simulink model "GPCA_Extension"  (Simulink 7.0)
settings: Solver=ode45  StartTime=0.0  StopTime=inf  RelTol=1e-3
PreLoadFcn:
  | GPCA_Bus_Def
InitFcn:
  | script
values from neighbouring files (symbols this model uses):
  GOutputEvents = [0 0 0 0 0 0 0 0 0 0 0 0 0 0 0 0 0 0 0 0 0]    [script.m]
  GProgrammedDoseRate = 0    [script.m]
  GProgrammedVTBI = 0    [script.m]
undefined symbols (not defined in the file or in its folder): BarcodeReader, patientReader, y1, y2, y3, y4, y5, y6
libraries: simulink x3
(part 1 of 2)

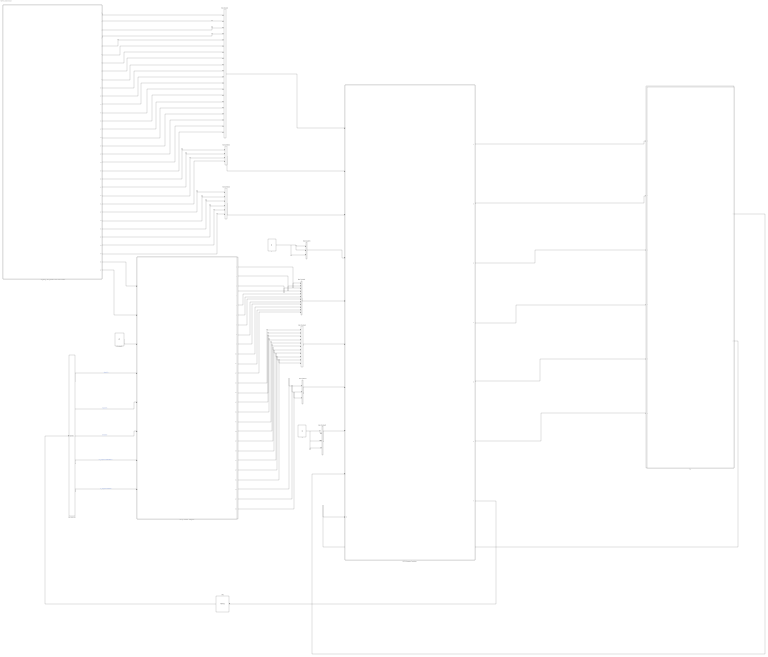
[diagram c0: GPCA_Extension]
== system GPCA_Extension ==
  1 : Constant  OutDataTypeMode=boolean  OutDataType=sfix(16)  OutScaling=2^0
  2 : Constant  Value=0  OutDataTypeMode=boolean  OutDataType=sfix(16)  OutScaling=2^0
  Bus Creator : BusCreator  Tag=DrugLIibraryInput  Description=Readings from the drug library  Inputs=20  UseBusObject=on
  Bus Creator1 : BusCreator  Description=Readings from the drug library  UseBusObject=on
  Bus Creator2 : BusCreator  Inputs=6  UseBusObject=on
  Bus Creator3 : BusCreator  Inputs=3  UseBusObject=on
  Bus Creator4 : BusCreator  Inputs=12  UseBusObject=on
  Bus Creator5 : BusCreator  Inputs=11  UseBusObject=on
  Bus Creator7 : BusCreator  Inputs=3  UseBusObject=on
  Bus Creator8 : BusCreator  Inputs=3  UseBusObject=on
  Bus Selector : BusSelector  OutputSignals=signal1,signal3,signal2,O_ProgrammedFlowRate,O_ProgrammedVTBI
  Constant5 : Constant  Value=0  OutDataType=sfix(16)  OutScaling=2^0
  Drug/Drug Library/Patient Information Reader : Subsystem
  GPCA Software Controller : Subsystem
  M2 : Memory  Orientation=left  InheritSampleTime=on
  Pump Controller Subsystem : Subsystem
  UI : Subsystem
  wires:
  Bus Creator/1 -> GPCA Software Controller/1(Drug Library Input)
  Bus Creator1/1 -> GPCA Software Controller/2(Patient Information Input)
  Bus Creator3/1 -> GPCA Software Controller/4(Environment Sensor Signals)
  Bus Creator4/1 -> GPCA Software Controller/5(Hardware Sensor Signals)
  Bus Creator7/1 -> GPCA Software Controller/7(Infusion Status Input)
  GPCA Software Controller/1(Drug Library Output) -> UI/1(Drug Lib)
  GPCA Software Controller/2(Patient Information Output) -> UI/2(Patient Info)
  GPCA Software Controller/4(Current State) -> UI/4(Current State)
  GPCA Software Controller/6(Alarming Condition) -> UI/6(Alarming Cond)
  GPCA Software Controller/3(Infusion Status Output) -> UI/3(Infusion Status)
  GPCA Software Controller/5(Drug Information Output) -> UI/5(Drug Info)
  1/1 -> Bus Creator8/1, Bus Creator8/2, Bus Creator8/3
  Bus Creator8/1 -> GPCA Software Controller/8(Pump Configuration Status Input)
  Bus Creator5/1 -> GPCA Software Controller/6(Infusion Sensor Signals)
  UI/2(Infusion Parameters) -> GPCA Software Controller/10(Infusion Parameters Input)
  UI/1(User Actions) -> GPCA Software Controller/9(User Actions)
  GPCA Software Controller/7(Infusion Instructions Output) -> M2/1
  Bus Selector/3 -> Pump Controller Subsystem/6(Infusion Paused)  "<signal2>"
  Bus Selector/2 -> Pump Controller Subsystem/5(Bolus Requested)  "<signal3>"
  Bus Selector/5 -> Pump Controller Subsystem/8(Programmed VTBI)  "<O_ProgrammedVTBI>"
  Bus Selector/1 -> Pump Controller Subsystem/4(Infusion In Progress)  "<signal1>"
  Bus Selector/4 -> Pump Controller Subsystem/7(Programmed Flow Rate)  "<O_ProgrammedFlowRate>"
  Constant5/1 -> Pump Controller Subsystem/3(New Bag Inserted)
  Drug/Drug Library/Patient Information Reader/32(Bolus Time) -> Pump Controller Subsystem/2(Bolus Time)
  Drug/Drug Library/Patient Information Reader/31(Bolus Volume) -> Pump Controller Subsystem/1(Bolus Volume)
  Bus Creator2/1 -> GPCA Software Controller/3(Drug Information Input)
  Drug/Drug Library/Patient Information Reader/30(drugVolumeUnit) -> Bus Creator2/6
  Drug/Drug Library/Patient Information Reader/29(drugDoseUnit) -> Bus Creator2/5
  Drug/Drug Library/Patient Information Reader/28(drugConcentration) -> Bus Creator2/4
  Drug/Drug Library/Patient Information Reader/27(drugDiluentVolume) -> Bus Creator2/3
  Drug/Drug Library/Patient Information Reader/26(drugDoseAmount) -> Bus Creator2/2
  Drug/Drug Library/Patient Information Reader/25(drugName) -> Bus Creator2/1
  Drug/Drug Library/Patient Information Reader/24(patientWeight) -> Bus Creator1/4
  Drug/Drug Library/Patient Information Reader/23(patientGender) -> Bus Creator1/3
  Drug/Drug Library/Patient Information Reader/22(patientAge) -> Bus Creator1/2
  Drug/Drug Library/Patient Information Reader/21(patientName) -> Bus Creator1/1
  Drug/Drug Library/Patient Information Reader/20(drugConcentrationLowerSoftLimit) -> Bus Creator/20
  Drug/Drug Library/Patient Information Reader/19(drugConcentrationLowerHardLimit) -> Bus Creator/19
  Drug/Drug Library/Patient Information Reader/18(drugConcentrationUpperSoftLimit) -> Bus Creator/18
  Drug/Drug Library/Patient Information Reader/17(drugConcentrationUpperHardLimit) -> Bus Creator/17
  Drug/Drug Library/Patient Information Reader/16(drugConcentrationTypical) -> Bus Creator/16
  Drug/Drug Library/Patient Information Reader/15(vtbiUnit) -> Bus Creator/15
  Drug/Drug Library/Patient Information Reader/14(vtbiLowerSoftLimit) -> Bus Creator/14
  Drug/Drug Library/Patient Information Reader/1(drugID) -> Bus Creator/1
  Drug/Drug Library/Patient Information Reader/2(amount) -> Bus Creator/2
  Drug/Drug Library/Patient Information Reader/3(diluentVolume) -> Bus Creator/3
  Drug/Drug Library/Patient Information Reader/4(doseRateTypical) -> Bus Creator/4
  Drug/Drug Library/Patient Information Reader/5(doseRateUpperHardLimit) -> Bus Creator/5
  Drug/Drug Library/Patient Information Reader/6(doseRateUpperSoftLimit) -> Bus Creator/6
  Drug/Drug Library/Patient Information Reader/7(doseRateLowerHardLimit) -> Bus Creator/7
  Drug/Drug Library/Patient Information Reader/8(doseRateLowerSoftLimit) -> Bus Creator/8
  Drug/Drug Library/Patient Information Reader/9(doseRateUnit) -> Bus Creator/9
  Drug/Drug Library/Patient Information Reader/10(vtbiTypical) -> Bus Creator/10
  Drug/Drug Library/Patient Information Reader/11(vtbiUpperHardLimit) -> Bus Creator/11
  Drug/Drug Library/Patient Information Reader/12(vtbiUpperSoftLimit) -> Bus Creator/12
  Drug/Drug Library/Patient Information Reader/13(vtbiLowerHardLimit) -> Bus Creator/13
  2/1 -> Bus Creator3/1, Bus Creator3/2, Bus Creator3/3
  Pump Controller Subsystem/1(Log Failure) -> Bus Creator4/1
  Pump Controller Subsystem/2(Watchdog Interrupt) -> Bus Creator4/2
  Pump Controller Subsystem/3(Door Open) -> Bus Creator4/3
  Pump Controller Subsystem/4(Battery Depleted) -> Bus Creator4/4
  Pump Controller Subsystem/5(Battery Low) -> Bus Creator4/5
  Pump Controller Subsystem/6(Battery Charge Error) -> Bus Creator4/6
  Pump Controller Subsystem/7(VoltOutRange) -> Bus Creator4/7
  Pump Controller Subsystem/8(CPU Error) -> Bus Creator4/8
  Pump Controller Subsystem/9(RTCError) -> Bus Creator4/9
  Pump Controller Subsystem/10(MemoryCorrupted) -> Bus Creator4/10
  Pump Controller Subsystem/11(PumpTooHot) -> Bus Creator4/11
  Pump Controller Subsystem/12(PumpOverheat) -> Bus Creator4/12
  Pump Controller Subsystem/13(EmptyReservoir) -> Bus Creator5/1
  Pump Controller Subsystem/14(LowReservoir) -> Bus Creator5/2
  Pump Controller Subsystem/15(Occlusion) -> Bus Creator5/3
  Pump Controller Subsystem/16(RateTooHigh) -> Bus Creator5/4
  Pump Controller Subsystem/17(RateTooLow) -> Bus Creator5/5
  Pump Controller Subsystem/18(LessThanKVO) -> Bus Creator5/6
  Pump Controller Subsystem/19(RateVary) -> Bus Creator5/7
  Pump Controller Subsystem/20(Flow Rate Above Pump Capacity Alarm) -> Bus Creator5/8
  Pump Controller Subsystem/21(PauseLong) -> Bus Creator5/9
  Pump Controller Subsystem/22(PauseTooLong) -> Bus Creator5/10
  Pump Controller Subsystem/23(Air In Line) -> Bus Creator5/11
  Pump Controller Subsystem/24(Bolus In Progress) -> Bus Creator7/1
  Pump Controller Subsystem/25(TotalVolumeInfused) -> Bus Creator7/2
  Pump Controller Subsystem/26(Current Volume) -> Bus Creator7/3
  M2/1 -> Bus Selector/1

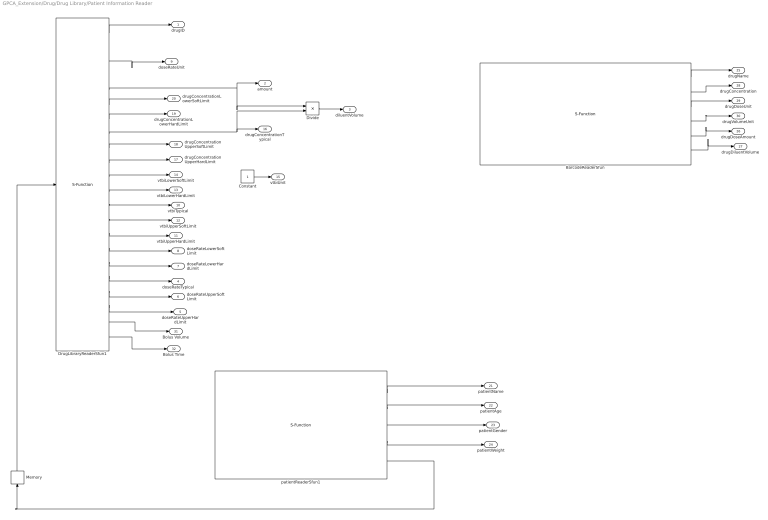
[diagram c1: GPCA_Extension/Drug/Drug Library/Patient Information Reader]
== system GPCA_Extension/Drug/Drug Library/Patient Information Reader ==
  BarcodeReaderSfun : S-Function  FunctionName=BarcodeReaderSfun  mask(Legacy Function){SFunctionSpec=BarcodeReader(uint32 y1[1], double y2[1], uint32 y3[1], uint32 y4[1], double y5[1], double y6[1]), ShowSpec=on}
      mask prompts: ShowSpec "Display function specification"
      mask help: This block allows the user to call the following C function(s) in Simulink: InitializeConditionsFcn: none StartFcn: openFile() OutputFcn: BarcodeReader(uint32 y1[1], double y2[1], uint32 y3[1], uint32 y4[1], double y5[1], double y6[1]) TerminateFcn: closeFile()
  Constant : Constant  OutDataTypeMode=uint32  OutDataType=sfix(16)  OutScaling=2^0
  Divide : Product  Inputs=*/  OutDataType=sfix(16)  OutScaling=2^-10
  DrugLibraryReaderSfun1 : S-Function  FunctionName=DrugLibraryReaderSfun  mask(Legacy Function){SFunctionSpec=DrugLibraryReader(uint32 u1[2], uint32 y1[1], uint32 y2[1], uint32 y3[1], uint32 y4[1], double  y5[1], double  y6[1], double  y7[1],double  y8[1],double  y9[1],double  y10[1],double  y11[1],double  y12[1], double  y13[1],double  y14[1],double  y15[1],double  y16[1],double  y17[1],double  y18[1],double  y19[1], double  y20[1],double  y21[1], uint32  y22[1]), ShowSpec=off}
      mask prompts: ShowSpec "Display function specification"
      mask help: This block allows the user to call the following C function(s) in Simulink: InitializeConditionsFcn: none StartFcn: openFile() OutputFcn: DrugLibraryReader(uint32 u1[2], uint32 y1[1], uint32 y2[1], uint32 y3[1], uint32 y4[1], double y5[1], double y6[1], double y7[1],double y8[1],double y9[1],double y10[1],double y11[1],double y12[1], double y13[1],double y14[1],double y15[1],double y16[1],double y17[1],double y18[1],double y19[1], double y20[1],double y21[1], uint32 y22[1]) TerminateFcn: closeFile()
  Memory : Memory  Orientation=up  InheritSampleTime=on
  patientReaderSfun1 : S-Function  FunctionName=patientReaderSfun  mask(Legacy Function){SFunctionSpec=patientReader(uint32 y1[1], uint32 y2[1], uint32 y3[1], uint32 y4[1], uint32 y5[2]), ShowSpec=on}
      mask prompts: ShowSpec "Display function specification"
      mask help: This block allows the user to call the following C function(s) in Simulink: InitializeConditionsFcn: randomizeSeed() StartFcn: openFile() OutputFcn: patientReader(uint32 y1[1], uint32 y2[1], uint32 y3[1], uint32 y4[1], uint32 y5[2]) TerminateFcn: closeFile()
  drugID : Outport  OutDataType=sfix(16)  OutScaling=2^0
  amount : Outport  Port=2  OutDataType=sfix(16)  OutScaling=2^0
  diluentVolume : Outport  Port=3  OutDataType=sfix(16)  OutScaling=2^0
  doseRateTypical : Outport  Port=4  OutDataType=sfix(16)  OutScaling=2^0
  doseRateUpperHardLimit : Outport  Port=5  OutDataType=sfix(16)  OutScaling=2^0
  doseRateUpperSoftLimit : Outport  Port=6  OutDataType=sfix(16)  OutScaling=2^0
  doseRateLowerHardLimit : Outport  Port=7  OutDataType=sfix(16)  OutScaling=2^0
  doseRateLowerSoftLimit : Outport  Port=8  OutDataType=sfix(16)  OutScaling=2^0
  doseRateUnit : Outport  Port=9  OutDataType=sfix(16)  OutScaling=2^0
  vtbiTypical : Outport  Port=10  OutDataType=sfix(16)  OutScaling=2^0
  vtbiUpperHardLimit : Outport  Port=11  OutDataType=sfix(16)  OutScaling=2^0
  vtbiUpperSoftLimit : Outport  Port=12  OutDataType=sfix(16)  OutScaling=2^0
  vtbiLowerHardLimit : Outport  Port=13  OutDataType=sfix(16)  OutScaling=2^0
  vtbiLowerSoftLimit : Outport  Port=14  OutDataType=sfix(16)  OutScaling=2^0
  vtbiUnit : Outport  Port=15  OutDataType=sfix(16)  OutScaling=2^0
  drugConcentrationTypical : Outport  Port=16  OutDataType=sfix(16)  OutScaling=2^0
  drugConcentrationUpperHardLimit : Outport  Port=17  OutDataType=sfix(16)  OutScaling=2^0
  drugConcentrationUpperSoftLimit : Outport  Port=18  OutDataType=sfix(16)  OutScaling=2^0
  drugConcentrationLowerHardLimit : Outport  Port=19  OutDataType=sfix(16)  OutScaling=2^0
  drugConcentrationLowerSoftLimit : Outport  Port=20  OutDataType=sfix(16)  OutScaling=2^0
  patientName : Outport  Port=21  OutDataType=sfix(16)  OutScaling=2^0
  patientAge : Outport  Port=22  OutDataType=sfix(16)  OutScaling=2^0
  patientGender : Outport  Port=23  OutDataType=sfix(16)  OutScaling=2^0
  patientWeight : Outport  Port=24  OutDataType=sfix(16)  OutScaling=2^0
  drugName : Outport  Port=25  OutDataType=sfix(16)  OutScaling=2^0
  drugDoseAmount : Outport  Port=26  OutDataType=sfix(16)  OutScaling=2^0
  drugDiluentVolume : Outport  Port=27  OutDataType=sfix(16)  OutScaling=2^0
  drugConcentration : Outport  Port=28  OutDataType=sfix(16)  OutScaling=2^0
  drugDoseUnit : Outport  Port=29  OutDataType=sfix(16)  OutScaling=2^0
  drugVolumeUnit : Outport  Port=30  OutDataType=sfix(16)  OutScaling=2^0
  Bolus Volume : Outport  Port=31  OutDataType=sfix(16)  OutScaling=2^0
  Bolus Time : Outport  Port=32  OutDataType=sfix(16)  OutScaling=2^0
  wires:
  patientReaderSfun1/5 -> Memory/1
  Memory/1 -> DrugLibraryReaderSfun1/1
  Divide/1 -> diluentVolume/1
  Constant/1 -> vtbiUnit/1
  patientReaderSfun1/1 -> patientName/1
  patientReaderSfun1/2 -> patientAge/1
  patientReaderSfun1/3 -> patientGender/1
  patientReaderSfun1/4 -> patientWeight/1
  BarcodeReaderSfun/1 -> drugName/1
  BarcodeReaderSfun/2 -> drugConcentration/1
  BarcodeReaderSfun/3 -> drugDoseUnit/1
  BarcodeReaderSfun/4 -> drugVolumeUnit/1
  BarcodeReaderSfun/5 -> drugDoseAmount/1
  BarcodeReaderSfun/6 -> drugDiluentVolume/1
  DrugLibraryReaderSfun1/1 -> drugID/1
  DrugLibraryReaderSfun1/5 -> amount/1, Divide/1
  DrugLibraryReaderSfun1/6 -> drugConcentrationLowerSoftLimit/1
  DrugLibraryReaderSfun1/7 -> drugConcentrationLowerHardLimit/1
  DrugLibraryReaderSfun1/8 -> drugConcentrationTypical/1, Divide/2
  DrugLibraryReaderSfun1/9 -> drugConcentrationUpperSoftLimit/1
  DrugLibraryReaderSfun1/10 -> drugConcentrationUpperHardLimit/1
  DrugLibraryReaderSfun1/11 -> vtbiLowerSoftLimit/1
  DrugLibraryReaderSfun1/12 -> vtbiLowerHardLimit/1
  DrugLibraryReaderSfun1/13 -> vtbiTypical/1
  DrugLibraryReaderSfun1/14 -> vtbiUpperSoftLimit/1
  DrugLibraryReaderSfun1/15 -> vtbiUpperHardLimit/1
  DrugLibraryReaderSfun1/16 -> doseRateLowerSoftLimit/1
  DrugLibraryReaderSfun1/17 -> doseRateLowerHardLimit/1
  DrugLibraryReaderSfun1/18 -> doseRateTypical/1
  DrugLibraryReaderSfun1/19 -> doseRateUpperSoftLimit/1
  DrugLibraryReaderSfun1/20 -> doseRateUpperHardLimit/1
  DrugLibraryReaderSfun1/3 -> doseRateUnit/1
  DrugLibraryReaderSfun1/21 -> Bolus Volume/1
  DrugLibraryReaderSfun1/22 -> Bolus Time/1

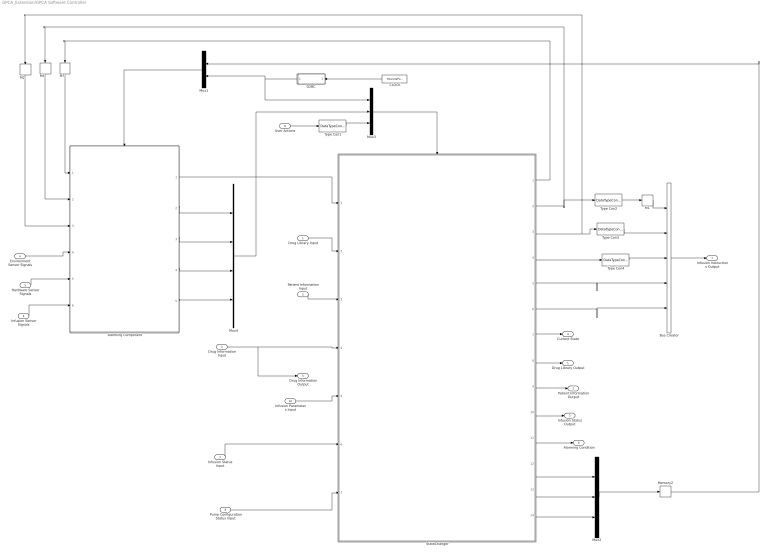
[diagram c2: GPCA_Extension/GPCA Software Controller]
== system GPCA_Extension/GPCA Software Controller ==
  Drug Library Input : Inport  OutDataType=sfix(16)  OutScaling=2^0
  Patient Information Input : Inport  Port=2  OutDataType=sfix(16)  OutScaling=2^0
  Drug Information Input : Inport  Port=3  OutDataType=sfix(16)  OutScaling=2^0
  Environment Sensor Signals : Inport  Port=4  OutDataType=sfix(16)  OutScaling=2^0
  Hardware Sensor Signals : Inport  Port=5  OutDataType=sfix(16)  OutScaling=2^0
  Infusion Sensor Signals : Inport  Port=6  OutDataType=sfix(16)  OutScaling=2^0
  Infusion Status Input : Inport  Port=7  OutDataType=sfix(16)  OutScaling=2^0
  Pump Configuration Status Input : Inport  Port=8  OutDataType=sfix(16)  OutScaling=2^0
  User Actions : Inport  Port=9  OutDataType=sfix(16)  OutScaling=2^0
  Infusion Parameters Input : Inport  Port=10  OutDataType=sfix(16)  OutScaling=2^0
  Alarming Component : Stateflow chart
  Bus Creator : BusCreator  Inputs=5  UseBusObject=on
  CLOCK : DiscretePulseGenerator  Orientation=left  PulseType=Time based  PulseWidth=50
  D2BC : Stateflow chart  Orientation=left
  M1 : Memory  InheritSampleTime=on
  M2 : Memory  Orientation=down  InheritSampleTime=on
  M4 : Memory  Orientation=down  InheritSampleTime=on
  M7 : Memory  Orientation=down  InheritSampleTime=on
  Memory2 : Memory  InheritSampleTime=on
  Mux1 : Mux  Orientation=left  Inputs=2
  Mux2 : Mux  Inputs=3
  Mux3 : Mux  Inputs=3
  Mux4 : Mux
  StateChanger : Stateflow chart
  Type Con1 : DataTypeConversion  OutDataTypeMode=boolean  OutDataType=sfix(16)  OutScaling=2^0
  Type Con2 : DataTypeConversion  OutDataType=sfix(16)  OutScaling=2^0
  Type Con3 : DataTypeConversion  OutDataType=sfix(16)  OutScaling=2^0
  Type Con4 : DataTypeConversion  OutDataType=sfix(16)  OutScaling=2^0
  Drug Library Output : Outport  OutDataType=sfix(16)  OutScaling=2^0
  Patient Information Output : Outport  Port=2  OutDataType=sfix(16)  OutScaling=2^0
  Infusion Status Output : Outport  Port=3  OutDataType=sfix(16)  OutScaling=2^0
  Current State : Outport  Port=4  OutDataType=sfix(16)  OutScaling=2^0
  Drug Information Output : Outport  Port=5  OutDataType=sfix(16)  OutScaling=2^0
  Alarming Condition : Outport  Port=6  OutDataType=sfix(16)  OutScaling=2^0
  Infusion Instructions Output : Outport  Port=7  OutDataType=sfix(16)  OutScaling=2^0
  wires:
  StateChanger/1(ClearCond) -> M7/1
  Mux3/1 -> StateChanger/Trigger
  Mux1/1 -> Alarming Component/Trigger
  StateChanger/2(O_InfusionInProgress) -> M4/1, Type Con2/1
  Alarming Component/1(ErrCond) -> StateChanger/1(ErrCond)
  User Actions/1 -> Type Con1/1
  StateChanger/12(E_Restart) -> Mux2/1
  StateChanger/13(E_AlarmClear) -> Mux2/2
  StateChanger/14(E_RequestToStart) -> Mux2/3
  Mux2/1 -> Memory2/1
  CLOCK/1 -> D2BC/1(u)
  D2BC/1(y) -> Mux1/2, Mux3/1
  Alarming Component/2(E_Alarm) -> Mux4/1
  Alarming Component/3(E_Warning) -> Mux4/2
  Alarming Component/4(E_Ready) -> Mux4/3
  Alarming Component/5(E_NotReady) -> Mux4/4
  Type Con1/1 -> Mux3/3
  Mux4/1 -> Mux3/2
  Type Con2/1 -> M1/1
  Memory2/1 -> Mux1/1
  Environment Sensor Signals/1 -> Alarming Component/4(envSenData)
  Hardware Sensor Signals/1 -> Alarming Component/5(hardwareSenData)
  Infusion Sensor Signals/1 -> Alarming Component/6(infuSenData)
  Drug Library Input/1 -> StateChanger/2(drugLibInfo)
  Patient Information Input/1 -> StateChanger/3(patientInfo)
  Drug Information Input/1 -> StateChanger/4(drugInfo), Drug Information Output/1
  Infusion Parameters Input/1 -> StateChanger/5(infuParameters)
  Infusion Status Input/1 -> StateChanger/6(infuStatus)
  Pump Configuration Status Input/1 -> StateChanger/7(pumpConfigData)
  StateChanger/11(O_AlarmCond) -> Alarming Condition/1
  StateChanger/7(O_CurrentState) -> Current State/1
  StateChanger/9(O_PatientInfo) -> Patient Information Output/1
  StateChanger/8(O_DrugLibInfo) -> Drug Library Output/1
  M1/1 -> Bus Creator/1
  StateChanger/3(O_InfusionPaused) -> M2/1, Type Con3/1
  Bus Creator/1 -> Infusion Instructions Output/1
  M7/1 -> Alarming Component/1(ClearCond)
  M4/1 -> Alarming Component/2(infusionInProgress)
  M2/1 -> Alarming Component/3(infusionPaused)
  StateChanger/4(O_BolusRequested) -> Type Con4/1
  StateChanger/5(O_ProgrammedVTBI) -> Bus Creator/4
  StateChanger/6(O_ProgrammedFlowRate) -> Bus Creator/5
  Type Con3/1 -> Bus Creator/2
  Type Con4/1 -> Bus Creator/3
  StateChanger/10(O_InfuStatus) -> Infusion Status Output/1

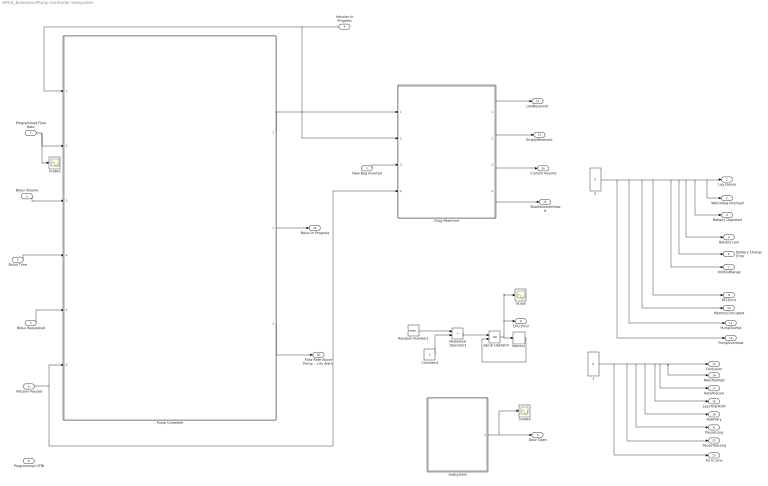
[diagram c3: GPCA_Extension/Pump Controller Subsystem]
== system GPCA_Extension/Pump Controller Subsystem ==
  Bolus Volume : Inport
  Bolus Time : Inport  Port=2
  New Bag Inserted : Inport  Port=3
  Infusion In Progress : Inport  Orientation=left  Port=4
  Bolus Requested : Inport  Port=5
  Infusion Paused : Inport  Port=6  OutDataType=sfix(16)  OutScaling=2^0
  Programmed Flow Rate : Inport  Port=7
  Programmed VTBI : Inport  Port=8
  1 : Constant  Value=0  OutDataTypeMode=boolean  OutDataType=sfix(16)  OutScaling=2^0
  2 : Constant  Value=0  OutDataTypeMode=boolean  OutDataType=sfix(16)  OutScaling=2^0
  Constant1 : Constant  Value=5  OutDataType=sfix(16)  OutScaling=2^0
  Drug Reservoir : Subsystem
  Logical Operator : Logic  Operator=OR  AllPortsSameDT=off  OutDataTypeMode=boolean
  Memory : Memory
  Pump Controller : Subsystem
  Random Number1 : RandomNumber  Mean=0.5
  Relational Operator1 : RelationalOperator  Operator=>  LogicOutDataTypeMode=boolean
  Scope : Scope
  Scope1 : Scope
  Scope2 : Scope
  Subsystem : Subsystem
  Log Failure : Outport  OutDataType=sfix(16)  OutScaling=2^0
  Watchdog Interrupt : Outport  Port=2  OutDataType=sfix(16)  OutScaling=2^0
  Door Open : Outport  Port=3  OutDataType=sfix(16)  OutScaling=2^0
  Battery Depleted : Outport  Port=4  OutDataType=sfix(16)  OutScaling=2^0
  Battery Low : Outport  Port=5  OutDataType=sfix(16)  OutScaling=2^0
  Battery Charge Error : Outport  Port=6  OutDataType=sfix(16)  OutScaling=2^0
  VoltOutRange : Outport  Port=7  OutDataType=sfix(16)  OutScaling=2^0
  CPU Error : Outport  Port=8  OutDataType=sfix(16)  OutScaling=2^0
  RTCError : Outport  Port=9  OutDataType=sfix(16)  OutScaling=2^0
  MemoryCorrupted : Outport  Port=10  OutDataType=sfix(16)  OutScaling=2^0
  PumpTooHot : Outport  Port=11  OutDataType=sfix(16)  OutScaling=2^0
  PumpOverheat : Outport  Port=12  OutDataType=sfix(16)  OutScaling=2^0
  EmptyReservoir : Outport  Port=13  OutDataType=sfix(16)  OutScaling=2^0
  LowReservoir : Outport  Port=14  OutDataType=sfix(16)  OutScaling=2^0
  Occlusion : Outport  Port=15  OutDataType=sfix(16)  OutScaling=2^0
  RateTooHigh : Outport  Port=16  OutDataType=sfix(16)  OutScaling=2^0
  RateTooLow : Outport  Port=17  OutDataType=sfix(16)  OutScaling=2^0
  LessThanKVO : Outport  Port=18  OutDataType=sfix(16)  OutScaling=2^0
  RateVary : Outport  Port=19  OutDataType=sfix(16)  OutScaling=2^0
  Flow Rate Above Pump Capacity Alarm : Outport  Port=20  OutDataType=sfix(16)  OutScaling=2^0
  PauseLong : Outport  Port=21  OutDataType=sfix(16)  OutScaling=2^0
  PauseTooLong : Outport  Port=22  OutDataType=sfix(16)  OutScaling=2^0
  Air In Line : Outport  Port=23  OutDataType=sfix(16)  OutScaling=2^0
  Bolus In Progress : Outport  Port=24  OutDataType=sfix(16)  OutScaling=2^0
  TotalVolumeInfused : Outport  Port=25  OutDataType=sfix(16)  OutScaling=2^0
  Current Volume : Outport  Port=26  OutDataType=sfix(16)  OutScaling=2^0
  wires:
  Bolus Requested/1 -> Pump Controller/5(Bolus Requested)
  Pump Controller/2(Bolus In Progress) -> Bolus In Progress/1
  Infusion Paused/1 -> Pump Controller/6(Infusion Paused), Drug Reservoir/4(Infusion Paused)
  New Bag Inserted/1 -> Drug Reservoir/3(New Bag Inserted)
  Drug Reservoir/3(Current Volume) -> Current Volume/1
  Drug Reservoir/2(DVA) -> EmptyReservoir/1
  Drug Reservoir/4(Total Volume Infused From Start) -> TotalVolumeInfused/1
  Infusion In Progress/1 -> Pump Controller/1(Infusion In Progress), Drug Reservoir/2(Infusion In Progress)
  Programmed Flow Rate/1 -> Pump Controller/2(Programmed Flow Rate), Scope1/1
  Drug Reservoir/1(LVW) -> LowReservoir/1
  Pump Controller/3(Flow Rate Above Pump Capacity Alarm) -> Flow Rate Above Pump Capacity Alarm/1
  Bolus Time/1 -> Pump Controller/4(Bolus Time)
  Bolus Volume/1 -> Pump Controller/3(Bolus Volume)
  2/1 -> RTCError/1, Battery Charge Error/1, Battery Low/1, Log Failure/1, Watchdog Interrupt/1, Battery Depleted/1, VoltOutRange/1, MemoryCorrupted/1, PumpTooHot/1, PumpOverheat/1
  1/1 -> RateTooLow/1, RateTooHigh/1, Occlusion/1, LessThanKVO/1, RateVary/1, PauseLong/1, PauseTooLong/1, Air In Line/1
  Pump Controller/1(Flow Rate) -> Drug Reservoir/1(Flow Rate)
  Random Number1/1 -> Relational Operator1/1
  Constant1/1 -> Relational Operator1/2
  Relational Operator1/1 -> Logical Operator/1
  Logical Operator/1 -> Memory/1, CPU Error/1, Scope/1
  Memory/1 -> Logical Operator/2
  Subsystem/1(Out1) -> Scope2/1, Door Open/1

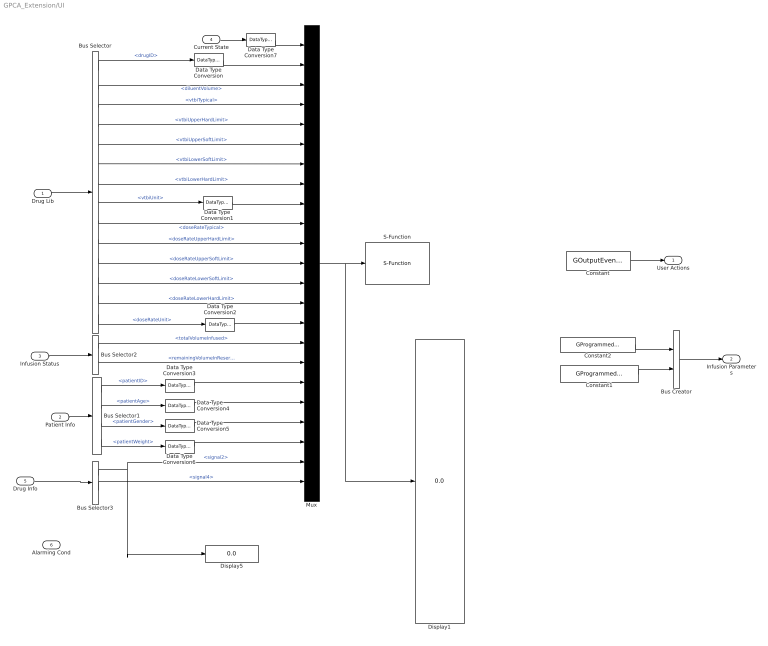
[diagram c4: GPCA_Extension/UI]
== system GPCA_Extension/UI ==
  Drug Lib : Inport  OutDataType=sfix(16)  OutScaling=2^0
  Patient Info : Inport  Port=2  OutDataType=sfix(16)  OutScaling=2^0
  Infusion Status : Inport  Port=3  OutDataType=sfix(16)  OutScaling=2^0
  Current State : Inport  Port=4  OutDataType=sfix(16)  OutScaling=2^0
  Drug Info : Inport  Port=5  OutDataType=sfix(16)  OutScaling=2^0
  Alarming Cond : Inport  Port=6  OutDataType=sfix(16)  OutScaling=2^0
  Bus Creator : BusCreator  Inputs=2  UseBusObject=on
  Bus Selector : BusSelector  OutputSignals=drugID,diluentVolume,vtbiTypical,vtbiUpperHardLimit,vtbiUpperSoftLimit,vtbiLowerSoftLimit,vtbiLowerHardLimit,vtbiUnit,doseRateTypical,doseRateUpperHardLimit,doseRateUpperSoftLimit,doseRateLowerSoftLimit,doseRateLowerHardLimit,doseRateUnit
  Bus Selector1 : BusSelector  OutputSignals=patientID,patientAge,patientGender,patientWeight
  Bus Selector2 : BusSelector  OutputSignals=totalVolumeInfused,remainingVolumeInReservoir
  Bus Selector3 : BusSelector  OutputSignals=signal2,signal4
  Constant : Constant  Value=GOutputEvents  OutDataType=sfix(16)  OutScaling=2^0
  Constant1 : Constant  Value=GProgrammedDoseRate  OutDataType=sfix(16)  OutScaling=2^0
  Constant2 : Constant  Value=GProgrammedVTBI  OutDataType=sfix(16)  OutScaling=2^0
  Data Type Conversion{,1..7} (8 alike) : DataTypeConversion  OutDataType=sfix(16)  OutScaling=2^0
  Display1 : Display
  Display5 : Display
  Mux : Mux  Inputs=23
  S-Function : S-Function  FunctionName=GPCA_UI_SFUN
  User Actions : Outport  OutDataType=sfix(16)  OutScaling=2^0
  Infusion Parameters : Outport  Port=2  OutDataType=sfix(16)  OutScaling=2^0
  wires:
  Current State/1 -> Data Type Conversion7/1
  Drug Lib/1 -> Bus Selector/1
  Bus Selector/1 -> Data Type Conversion/1  "<drugID>"
  Bus Selector/2 -> Mux/3  "<diluentVolume>"
  Bus Selector/3 -> Mux/4  "<vtbiTypical>"
  Bus Selector/4 -> Mux/5  "<vtbiUpperHardLimit>"
  Bus Selector/5 -> Mux/6  "<vtbiUpperSoftLimit>"
  Bus Selector/6 -> Mux/7  "<vtbiLowerSoftLimit>"
  Bus Selector/7 -> Mux/8  "<vtbiLowerHardLimit>"
  Bus Selector/8 -> Data Type Conversion1/1  "<vtbiUnit>"
  Bus Selector/9 -> Mux/10  "<doseRateTypical>"
  Bus Selector/10 -> Mux/11  "<doseRateUpperHardLimit>"
  Bus Selector/11 -> Mux/12  "<doseRateUpperSoftLimit>"
  Bus Selector/12 -> Mux/13  "<doseRateLowerSoftLimit>"
  Bus Selector/13 -> Mux/14  "<doseRateLowerHardLimit>"
  Bus Selector/14 -> Data Type Conversion2/1  "<doseRateUnit>"
  Patient Info/1 -> Bus Selector1/1
  Bus Selector1/1 -> Data Type Conversion3/1  "<patientID>"
  Bus Selector1/2 -> Data Type Conversion4/1  "<patientAge>"
  Bus Selector1/3 -> Data Type Conversion5/1  "<patientGender>"
  Bus Selector1/4 -> Data Type Conversion6/1  "<patientWeight>"
  Bus Selector3/1 -> Mux/22, Display5/1  "<signal2>"
  Bus Selector3/2 -> Mux/23  "<signal4>"
  Data Type Conversion/1 -> Mux/2
  Data Type Conversion1/1 -> Mux/9
  Data Type Conversion2/1 -> Mux/15
  Data Type Conversion3/1 -> Mux/18
  Data Type Conversion4/1 -> Mux/19
  Data Type Conversion5/1 -> Mux/20
  Data Type Conversion6/1 -> Mux/21
  Infusion Status/1 -> Bus Selector2/1
  Drug Info/1 -> Bus Selector3/1
  Constant/1 -> User Actions/1
  Constant2/1 -> Bus Creator/1
  Constant1/1 -> Bus Creator/2
  Bus Creator/1 -> Infusion Parameters/1
  Bus Selector2/1 -> Mux/16  "<totalVolumeInfused>"
  Bus Selector2/2 -> Mux/17  "<remainingVolumeInReservoir>"
  Data Type Conversion7/1 -> Mux/1
  Mux/1 -> S-Function/1, Display1/1

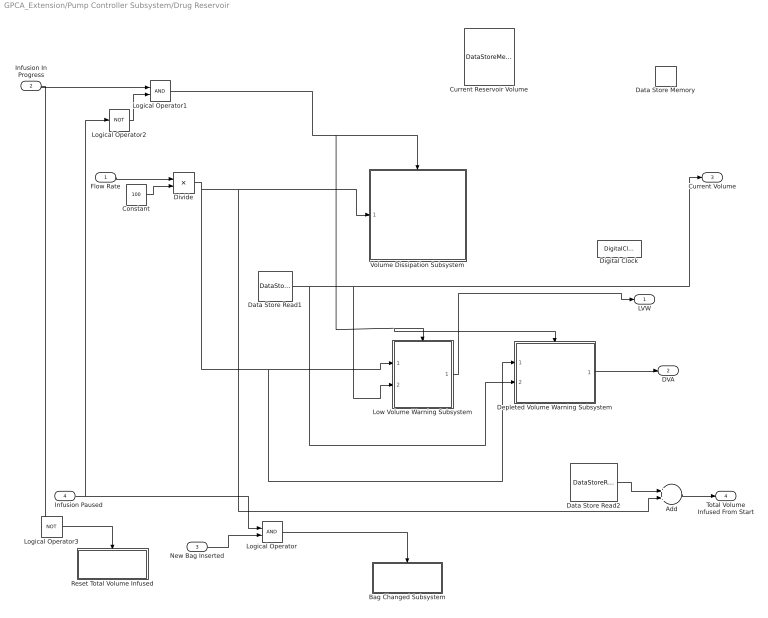
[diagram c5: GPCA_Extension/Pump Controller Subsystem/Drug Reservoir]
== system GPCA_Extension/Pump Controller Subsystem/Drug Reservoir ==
  Flow Rate : Inport
  Infusion In Progress : Inport  Port=2  OutDataType=sfix(16)  OutScaling=2^0
  New Bag Inserted : Inport  Port=3  OutDataType=sfix(16)  OutScaling=2^0
  Infusion Paused : Inport  Port=4  OutDataType=sfix(16)  OutScaling=2^0
  Add : Sum  OutDataType=sfix(16)  OutScaling=2^-10
  Bag Changed Subsystem : Subsystem  TreatAsAtomicUnit=on
  Constant : Constant  Value=100  OutDataType=sfix(16)  OutScaling=2^0
  Current Reservoir Volume : DataStoreMemory  DataStoreName=VolumeRes  InitialValue=2500  OutDataType=sfix(16)  OutScaling=2^0
  Data Store Memory : DataStoreMemory  DataStoreName=TVI  OutDataType=sfix(16)  OutScaling=2^0
  Data Store Read1 : DataStoreRead  DataStoreName=VolumeRes  SampleTime=-1
  Data Store Read2 : DataStoreRead  DataStoreName=TVI  SampleTime=-1
  Depleted Volume Warning Subsystem : Subsystem
  Digital Clock : DigitalClock
  Divide : Product  Inputs=*/  OutDataType=sfix(16)  OutScaling=2^-10
  Logical Operator : Logic  AllPortsSameDT=off  OutDataTypeMode=boolean
  Logical Operator1 : Logic  AllPortsSameDT=off  OutDataTypeMode=boolean
  Logical Operator2 : Logic  Operator=NOT  AllPortsSameDT=off  OutDataTypeMode=boolean
  Logical Operator3 : Logic  Operator=NOT  AllPortsSameDT=off  OutDataTypeMode=boolean
  Low Volume Warning Subsystem : Subsystem
  Reset Total Volume Infused : Subsystem  TreatAsAtomicUnit=on
  Volume Dissipation Subsystem : Subsystem
  LVW : Outport  OutDataType=sfix(16)  OutScaling=2^0
  DVA : Outport  Port=2  OutDataType=sfix(16)  OutScaling=2^0
  Current Volume : Outport  Port=3  OutDataType=sfix(16)  OutScaling=2^0
  Total Volume Infused From Start : Outport  Port=4  OutDataType=sfix(16)  OutScaling=2^0
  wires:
  Divide/1 -> Low Volume Warning Subsystem/1(Flow Rate), Depleted Volume Warning Subsystem/1(Flow Rate), Volume Dissipation Subsystem/1(Flow Rate), Add/2
  Logical Operator1/1 -> Volume Dissipation Subsystem/Enable, Low Volume Warning Subsystem/Enable, Depleted Volume Warning Subsystem/Enable
  Depleted Volume Warning Subsystem/1(DVA) -> DVA/1
  Low Volume Warning Subsystem/1(LVW) -> LVW/1
  Data Store Read1/1 -> Depleted Volume Warning Subsystem/2(Volume), Low Volume Warning Subsystem/2(Volume), Current Volume/1
  Infusion Paused/1 -> Logical Operator/1, Logical Operator2/1
  New Bag Inserted/1 -> Logical Operator/2
  Logical Operator/1 -> Bag Changed Subsystem/Enable
  Data Store Read2/1 -> Add/1
  Add/1 -> Total Volume Infused From Start/1
  Flow Rate/1 -> Divide/1
  Constant/1 -> Divide/2
  Infusion In Progress/1 -> Logical Operator1/1, Logical Operator3/1
  Logical Operator2/1 -> Logical Operator1/2
  Logical Operator3/1 -> Reset Total Volume Infused/Enable

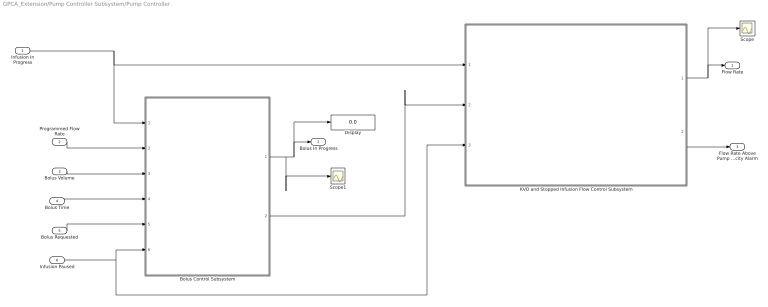
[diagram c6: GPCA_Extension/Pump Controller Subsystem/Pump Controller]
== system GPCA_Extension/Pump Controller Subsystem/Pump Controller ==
  Infusion In Progress : Inport  OutDataType=sfix(16)  OutScaling=2^0
  Programmed Flow Rate : Inport  Port=2  OutDataType=sfix(16)  OutScaling=2^0
  Bolus Volume : Inport  Port=3  OutDataType=sfix(16)  OutScaling=2^0
  Bolus Time : Inport  Port=4  OutDataType=sfix(16)  OutScaling=2^0
  Bolus Requested : Inport  Port=5  OutDataType=sfix(16)  OutScaling=2^0
  Infusion Paused : Inport  Port=6  OutDataType=sfix(16)  OutScaling=2^0
  Bolus Control Subsystem : Subsystem
  Display : Display
  KVO and Stopped Infusion Flow Control Subsystem : Subsystem
  Scope : Scope
  Scope1 : Scope
  Flow Rate : Outport
  Bolus In Progress : Outport  Port=2
  Flow Rate Above Pump Capacity Alarm : Outport  Port=3  OutDataType=sfix(16)  OutScaling=2^0
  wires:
  Infusion In Progress/1 -> KVO and Stopped Infusion Flow Control Subsystem/1(Infusion In Progress), Bolus Control Subsystem/1(Infusion In Progress)
  Programmed Flow Rate/1 -> Bolus Control Subsystem/2(Programmed Flow Rate)
  Bolus Requested/1 -> Bolus Control Subsystem/5(Bolus Requested)
  Bolus Volume/1 -> Bolus Control Subsystem/3(Bolus Volume)
  Bolus Time/1 -> Bolus Control Subsystem/4(Bolus Time)
  Bolus Control Subsystem/1(" Bolus In Progress") -> Scope1/1, Bolus In Progress/1, Display/1
  Infusion Paused/1 -> Bolus Control Subsystem/6(Infusion Paused), KVO and Stopped Infusion Flow Control Subsystem/3(Infusion Paused)
  Bolus Control Subsystem/2(Flow Rate) -> KVO and Stopped Infusion Flow Control Subsystem/2(Flow Rate from Bolus Subsystem)
  KVO and Stopped Infusion Flow Control Subsystem/1(Flow Rate) -> Flow Rate/1, Scope/1
  KVO and Stopped Infusion Flow Control Subsystem/2(" Flow Rate Above Pump Capacity Alarm") -> Flow Rate Above Pump Capacity Alarm/1

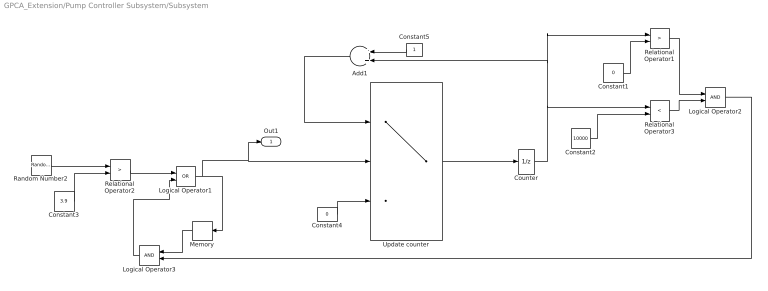
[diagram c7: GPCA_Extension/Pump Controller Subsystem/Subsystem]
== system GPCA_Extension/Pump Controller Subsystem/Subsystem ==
  Add1 : Sum  Orientation=left  OutDataType=sfix(16)  OutScaling=2^-10
  Constant1 : Constant  Value=0  OutDataType=sfix(16)  OutScaling=2^0
  Constant2 : Constant  Value=10000  OutDataType=sfix(16)  OutScaling=2^0
  Constant3 : Constant  Value=3.9  OutDataType=sfix(16)  OutScaling=2^0
  Constant4 : Constant  Value=0  OutDataType=sfix(16)  OutScaling=2^0
  Constant5 : Constant  Orientation=left  OutDataType=sfix(16)  OutScaling=2^0
  Counter : UnitDelay
  Logical Operator1 : Logic  Operator=OR  AllPortsSameDT=off  OutDataTypeMode=boolean
  Logical Operator2 : Logic  AllPortsSameDT=off  OutDataTypeMode=boolean
  Logical Operator3 : Logic  Orientation=left  AllPortsSameDT=off  OutDataTypeMode=boolean
  Memory : Memory  Orientation=left
  Random Number2 : RandomNumber  Mean=0.5
  Relational Operator1 : RelationalOperator  Operator=>  LogicOutDataTypeMode=boolean
  Relational Operator2 : RelationalOperator  Operator=>  LogicOutDataTypeMode=boolean
  Relational Operator3 : RelationalOperator  Operator=<  LogicOutDataTypeMode=boolean
  Update counter : Switch  Threshold=1  OutDataType=sfix(16)  OutScaling=2^0
  Out1 : Outport  OutDataType=sfix(16)  OutScaling=2^0
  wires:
  Random Number2/1 -> Relational Operator2/1
  Constant3/1 -> Relational Operator2/2
  Relational Operator2/1 -> Logical Operator1/1
  Logical Operator1/1 -> Memory/1, Update counter/2, Out1/1
  Add1/1 -> Update counter/1
  Constant5/1 -> Add1/1
  Counter/1 -> Relational Operator3/1, Add1/2, Relational Operator1/1
  Update counter/1 -> Counter/1
  Constant4/1 -> Update counter/3
  Constant2/1 -> Relational Operator3/2
  Relational Operator3/1 -> Logical Operator2/2
  Constant1/1 -> Relational Operator1/2
  Relational Operator1/1 -> Logical Operator2/1
  Memory/1 -> Logical Operator3/1
  Logical Operator2/1 -> Logical Operator3/2
  Logical Operator3/1 -> Logical Operator1/2

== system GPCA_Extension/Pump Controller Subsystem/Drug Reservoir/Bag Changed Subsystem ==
  Enable : EnablePort
  Constant : Constant  Value=10  OutDataType=sfix(16)  OutScaling=2^0
  Data Store Write : DataStoreWrite  DataStoreName=VolumeRes  SampleTime=-1
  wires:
  Constant/1 -> Data Store Write/1

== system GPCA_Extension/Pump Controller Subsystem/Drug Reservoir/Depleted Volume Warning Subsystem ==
  Flow Rate : Inport  OutDataType=sfix(16)  OutScaling=2^0
  Volume : Inport  Port=2  OutDataType=sfix(16)  OutScaling=2^0
  Enable : EnablePort
  Compare To Constant : simulink/Logic and Bit Operations/Compare To Constant  SystemSampleTime=-1  relop=<=  const=5  LogicOutDataTypeMode=boolean  ZeroCross=off
  Divide : Product  Inputs=*/  OutDataType=sfix(16)  OutScaling=2^-10
  DVA : Outport  OutDataType=sfix(16)  OutScaling=2^0
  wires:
  Volume/1 -> Divide/1
  Flow Rate/1 -> Divide/2
  Divide/1 -> Compare To Constant/1
  Compare To Constant/1 -> DVA/1

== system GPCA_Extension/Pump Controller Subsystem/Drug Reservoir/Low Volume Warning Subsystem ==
  Flow Rate : Inport  OutDataType=sfix(16)  OutScaling=2^0
  Volume : Inport  Port=2  OutDataType=sfix(16)  OutScaling=2^0
  Enable : EnablePort
  Compare To Constant : simulink/Logic and Bit Operations/Compare To Constant  SystemSampleTime=-1  relop=<=  const=15  LogicOutDataTypeMode=boolean  ZeroCross=off
  Compare To Constant1 : simulink/Logic and Bit Operations/Compare To Constant  SystemSampleTime=-1  relop=>  const=5  LogicOutDataTypeMode=boolean  ZeroCross=off
  Divide : Product  Inputs=*/  OutDataType=sfix(16)  OutScaling=2^-10
  Logical Operator : Logic  AllPortsSameDT=off  OutDataTypeMode=boolean
  LVW : Outport  OutDataType=sfix(16)  OutScaling=2^0
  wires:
  Volume/1 -> Divide/1
  Flow Rate/1 -> Divide/2
  Divide/1 -> Compare To Constant/1, Compare To Constant1/1
  Compare To Constant1/1 -> Logical Operator/2
  Compare To Constant/1 -> Logical Operator/1
  Logical Operator/1 -> LVW/1

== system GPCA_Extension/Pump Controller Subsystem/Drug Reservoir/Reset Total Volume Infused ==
  Enable : EnablePort
  Constant : Constant  Value=0  OutDataType=sfix(16)  OutScaling=2^0
  Data Store Write : DataStoreWrite  DataStoreName=TVI  SampleTime=-1
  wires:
  Constant/1 -> Data Store Write/1

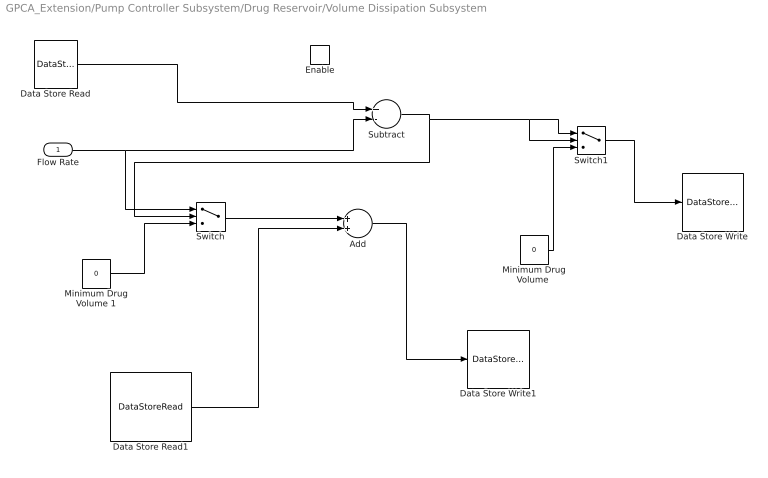
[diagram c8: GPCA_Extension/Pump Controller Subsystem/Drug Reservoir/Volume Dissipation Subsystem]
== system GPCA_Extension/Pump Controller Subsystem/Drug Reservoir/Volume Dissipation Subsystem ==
  Flow Rate : Inport  OutDataType=sfix(16)  OutScaling=2^0
  Enable : EnablePort
  Add : Sum  OutDataType=sfix(16)  OutScaling=2^-10
  Data Store Read : DataStoreRead  DataStoreName=VolumeRes  SampleTime=-1
  Data Store Read1 : DataStoreRead  DataStoreName=TVI  SampleTime=-1
  Data Store Write : DataStoreWrite  DataStoreName=VolumeRes  SampleTime=-1
  Data Store Write1 : DataStoreWrite  DataStoreName=TVI  SampleTime=-1
  "Minimum Drug Volume " : Constant  Value=0  OutDataTypeMode=double  OutDataType=sfix(16)  OutScaling=2^0
  Minimum Drug Volume 1 : Constant  Value=0  OutDataTypeMode=double  OutDataType=sfix(16)  OutScaling=2^0
  Subtract : Sum  Inputs=+-  OutDataType=sfix(16)  OutScaling=2^-10
  Switch : Switch  OutDataType=sfix(16)  OutScaling=2^0
  Switch1 : Switch  OutDataType=sfix(16)  OutScaling=2^0
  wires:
  Data Store Read/1 -> Subtract/1
  Flow Rate/1 -> Subtract/2, Switch/1
  Data Store Read1/1 -> Add/2
  Add/1 -> Data Store Write1/1
  Subtract/1 -> Switch/2, Switch1/1, Switch1/2
  Minimum Drug Volume 1/1 -> Switch/3
  Switch/1 -> Add/1
  "Minimum Drug Volume "/1 -> Switch1/3
  Switch1/1 -> Data Store Write/1

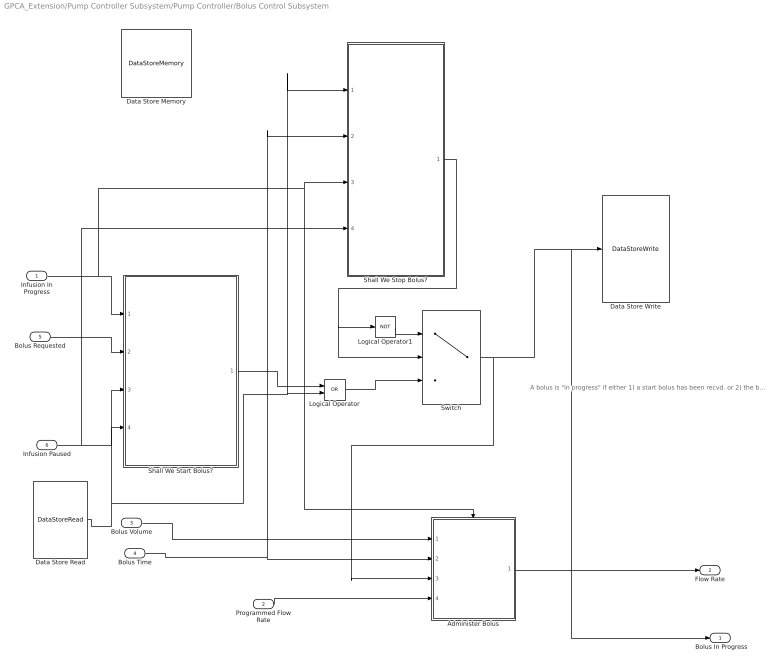
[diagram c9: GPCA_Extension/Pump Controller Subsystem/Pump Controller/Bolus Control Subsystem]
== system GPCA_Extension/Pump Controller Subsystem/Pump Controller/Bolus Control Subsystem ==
  note: A bolus is "in progress" if either 1) a start bolus has been recvd. or 2) the bolus was in progress in the preceeding simulation time. The only way a bolus that is in progress can become de-activated is if the bolus timer expires or if infusion is no longer in progress (can happen due to an alarm or user input). The switch block encodes this logic. As long as "Shall we Stop Bolus" outputs 0 (i.e. the bolus timer has not expired), the switch block outputs the value of "Start Bolus" OR "Bolus In Progress in Previous Step". As soon as "Shall We Stop Bolus" outputs 1, the switch outputs 0.
  Infusion In Progress : Inport  OutDataType=sfix(16)  OutScaling=2^0
  Programmed Flow Rate : Inport  Port=2  OutDataType=sfix(16)  OutScaling=2^0
  Bolus Volume : Inport  Port=3  OutDataType=sfix(16)  OutScaling=2^0
  Bolus Time : Inport  Port=4  OutDataType=sfix(16)  OutScaling=2^0
  Bolus Requested : Inport  Port=5  OutDataType=sfix(16)  OutScaling=2^0
  Infusion Paused : Inport  Port=6  OutDataType=sfix(16)  OutScaling=2^0
  Administer Bolus : Subsystem
  Data Store Memory : DataStoreMemory  DataStoreName=BolusInProgress  DataType=boolean  OutDataType=sfix(16)  OutScaling=2^0
  Data Store Read : DataStoreRead  DataStoreName=BolusInProgress  SampleTime=-1
  Data Store Write : DataStoreWrite  DataStoreName=BolusInProgress  SampleTime=-1
  Logical Operator : Logic  Operator=OR  AllPortsSameDT=off  OutDataTypeMode=boolean
  Logical Operator1 : Logic  Operator=NOT  AllPortsSameDT=off  OutDataTypeMode=boolean
  Shall We Start Bolus? : Subsystem
  Shall We Stop Bolus? : Subsystem
  Switch : Switch  Criteria=u2 ~= 0  OutDataType=sfix(16)  OutScaling=2^0
  " Bolus In Progress" : Outport  OutDataType=sfix(16)  OutScaling=2^0
  Flow Rate : Outport  Port=2  OutDataType=sfix(16)  OutScaling=2^0
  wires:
  Infusion In Progress/1 -> Shall We Start Bolus?/1(Infusion In Progress), Shall We Stop Bolus?/3(Infusion In Progress), Administer Bolus/Enable
  Bolus Requested/1 -> Shall We Start Bolus?/2(Bolus Requested)
  Data Store Read/1 -> Shall We Start Bolus?/3(Bolus In Progress), Logical Operator/2, Shall We Stop Bolus?/1(IsBolusInProgress)
  Bolus Volume/1 -> Administer Bolus/1(Bolus Volume)
  Bolus Time/1 -> Administer Bolus/2(Bolus Time), Shall We Stop Bolus?/2(Bolus Time)
  Programmed Flow Rate/1 -> Administer Bolus/4(Programmed Flow Rate)
  Administer Bolus/1(Out1) -> Flow Rate/1
  Switch/1 -> Administer Bolus/3(Bolus In Progress), Data Store Write/1, " Bolus In Progress"/1
  Shall We Start Bolus?/1(Start Bolus) -> Logical Operator/1
  Shall We Stop Bolus?/1(Stop Bolus) -> Switch/2, Logical Operator1/1
  Logical Operator1/1 -> Switch/1
  Infusion Paused/1 -> Shall We Start Bolus?/4(Infusion Paused), Shall We Stop Bolus?/4(Infusion Paused)
  Logical Operator/1 -> Switch/3

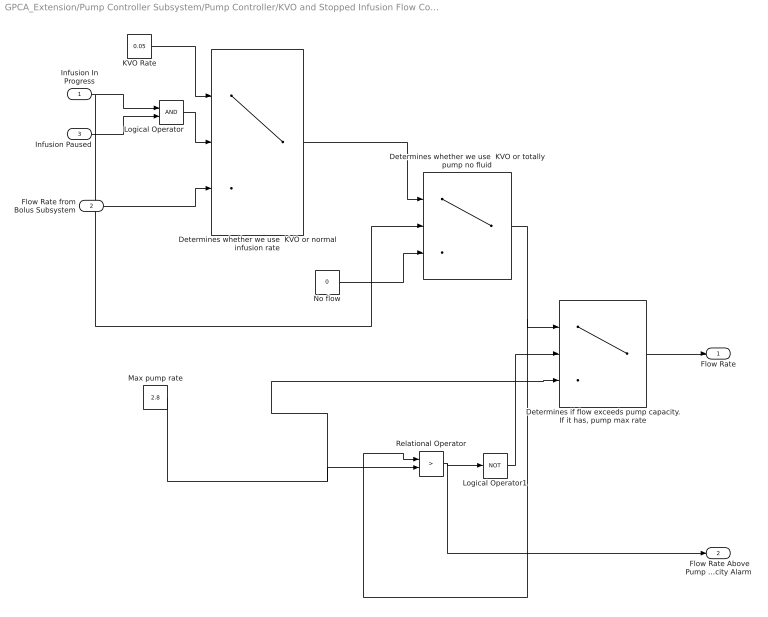
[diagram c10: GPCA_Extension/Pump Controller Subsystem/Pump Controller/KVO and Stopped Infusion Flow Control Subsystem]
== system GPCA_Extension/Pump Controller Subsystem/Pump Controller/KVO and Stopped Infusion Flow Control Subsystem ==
  Infusion In Progress : Inport
  Flow Rate from Bolus Subsystem : Inport  Port=2
  Infusion Paused : Inport  Port=3
  "Determines if flow exceeds pump capacity. If it has, pump max rate" : Switch  Criteria=u2 ~= 0  OutDataType=sfix(16)  OutScaling=2^0
  Determines whether we use  KVO or normal infusion rate : Switch  Criteria=u2 ~= 0  OutDataType=sfix(16)  OutScaling=2^0
  Determines whether we use  KVO or totally pump no fluid : Switch  Criteria=u2 ~= 0  OutDataType=sfix(16)  OutScaling=2^0
  KVO Rate : Constant  Value=0.05  OutDataType=sfix(16)  OutScaling=2^0
  Logical Operator : Logic  AllPortsSameDT=off  OutDataTypeMode=boolean
  Logical Operator1 : Logic  Operator=NOT  AllPortsSameDT=off  OutDataTypeMode=boolean
  Max pump rate : Constant  Value=2.8  OutDataType=sfix(16)  OutScaling=2^0
  No flow : Constant  Value=0  OutDataType=sfix(16)  OutScaling=2^0
  Relational Operator : RelationalOperator  Operator=>  LogicOutDataTypeMode=boolean
  Flow Rate : Outport
  " Flow Rate Above Pump Capacity Alarm" : Outport  Port=2  OutDataType=sfix(16)  OutScaling=2^0
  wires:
  KVO Rate/1 -> Determines whether we use  KVO or normal infusion rate/1
  Flow Rate from Bolus Subsystem/1 -> Determines whether we use  KVO or normal infusion rate/3
  Infusion In Progress/1 -> Logical Operator/1, Determines whether we use  KVO or totally pump no fluid/2
  Infusion Paused/1 -> Logical Operator/2
  Logical Operator/1 -> Determines whether we use  KVO or normal infusion rate/2
  Determines whether we use  KVO or normal infusion rate/1 -> Determines whether we use  KVO or totally pump no fluid/1
  No flow/1 -> Determines whether we use  KVO or totally pump no fluid/3
  "Determines if flow exceeds pump capacity. If it has, pump max rate"/1 -> Flow Rate/1
  Determines whether we use  KVO or totally pump no fluid/1 -> "Determines if flow exceeds pump capacity. If it has, pump max rate"/1, Relational Operator/1
  Max pump rate/1 -> "Determines if flow exceeds pump capacity. If it has, pump max rate"/3, Relational Operator/2
  Relational Operator/1 -> Logical Operator1/1, " Flow Rate Above Pump Capacity Alarm"/1
  Logical Operator1/1 -> "Determines if flow exceeds pump capacity. If it has, pump max rate"/2

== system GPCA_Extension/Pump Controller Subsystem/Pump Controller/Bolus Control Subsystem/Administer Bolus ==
  Bolus Volume : Inport  OutDataType=sfix(16)  OutScaling=2^0
  Bolus Time : Inport  Port=2  OutDataType=sfix(16)  OutScaling=2^0
  Bolus In Progress : Inport  Port=3
  Programmed Flow Rate : Inport  Port=4
  Enable : EnablePort
  Divide : Product  Inputs=*/  OutDataType=sfix(16)  OutScaling=2^-10
  Switch : Switch  Criteria=u2 ~= 0  OutDataType=sfix(16)  OutScaling=2^0
  Out1 : Outport
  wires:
  Bolus Volume/1 -> Divide/1
  Bolus Time/1 -> Divide/2
  Divide/1 -> Switch/1
  Bolus In Progress/1 -> Switch/2
  Switch/1 -> Out1/1
  Programmed Flow Rate/1 -> Switch/3

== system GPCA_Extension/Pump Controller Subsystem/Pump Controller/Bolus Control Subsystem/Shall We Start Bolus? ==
  Infusion In Progress : Inport  OutDataType=sfix(16)  OutScaling=2^0
  Bolus Requested : Inport  Port=2  OutDataType=sfix(16)  OutScaling=2^0
  Bolus In Progress : Inport  Port=3  OutDataType=sfix(16)  OutScaling=2^0
  Infusion Paused : Inport  Port=4  OutDataType=sfix(16)  OutScaling=2^0
  Logical Operator1 : Logic  Operator=NOT  AllPortsSameDT=off  OutDataTypeMode=boolean
  Logical Operator2 : Logic  Inputs=4  OutDataTypeMode=boolean
  Logical Operator3 : Logic  Operator=NOT  AllPortsSameDT=off  OutDataTypeMode=boolean
  Start Bolus : Outport  OutDataType=sfix(16)  OutScaling=2^0
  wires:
  Bolus Requested/1 -> Logical Operator2/2
  Bolus In Progress/1 -> Logical Operator1/1
  Infusion In Progress/1 -> Logical Operator2/1
  Logical Operator1/1 -> Logical Operator2/3
  Logical Operator2/1 -> Start Bolus/1
  Logical Operator3/1 -> Logical Operator2/4
  Infusion Paused/1 -> Logical Operator3/1

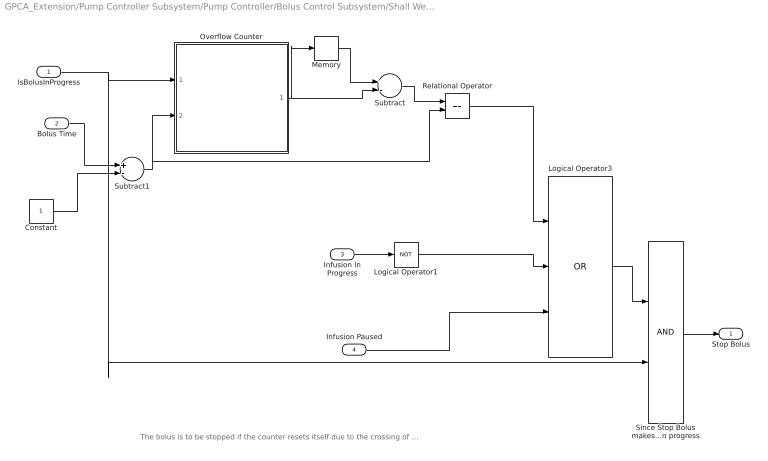
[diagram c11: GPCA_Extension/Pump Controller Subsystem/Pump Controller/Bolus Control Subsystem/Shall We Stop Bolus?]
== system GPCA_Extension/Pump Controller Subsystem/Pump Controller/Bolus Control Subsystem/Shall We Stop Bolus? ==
  note: The bolus is to be stopped if the counter resets itself due to the crossing of the upper limit. The memory block and the subtract block detects if the output of the counter fell from "Upper limit" to "zero"
  IsBolusInProgress : Inport
  Bolus Time : Inport  Port=2
  Infusion In Progress : Inport  Port=3  OutDataType=sfix(16)  OutScaling=2^0
  Infusion Paused : Inport  Port=4  OutDataType=sfix(16)  OutScaling=2^0
  Constant : Constant  OutDataType=sfix(16)  OutScaling=2^0
  Logical Operator1 : Logic  Operator=NOT  AllPortsSameDT=off  OutDataTypeMode=boolean
  Logical Operator3 : Logic  Operator=OR  Inputs=3  AllPortsSameDT=off  OutDataTypeMode=boolean
  Memory : Memory  InheritSampleTime=on
  Overflow Counter : Subsystem
  Relational Operator : RelationalOperator  Operator===  LogicOutDataTypeMode=boolean
  Since Stop Bolus makes sense only when there was bolus in progress : Logic  AllPortsSameDT=off  OutDataTypeMode=boolean
  Subtract : Sum  Inputs=+-  OutDataType=sfix(16)  OutScaling=2^-10
  Subtract1 : Sum  Inputs=+-  OutDataType=sfix(16)  OutScaling=2^-10
  Stop Bolus : Outport
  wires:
  Overflow Counter/1(Out1) -> Memory/1, Subtract/2
  IsBolusInProgress/1 -> Overflow Counter/1(Keep Running), Since Stop Bolus makes sense only when there was bolus in progress/2
  Memory/1 -> Subtract/1
  Subtract/1 -> Relational Operator/1
  Relational Operator/1 -> Logical Operator3/1
  Infusion In Progress/1 -> Logical Operator1/1
  Logical Operator1/1 -> Logical Operator3/2
  Infusion Paused/1 -> Logical Operator3/3
  Since Stop Bolus makes sense only when there was bolus in progress/1 -> Stop Bolus/1
  Logical Operator3/1 -> Since Stop Bolus makes sense only when there was bolus in progress/1
  Bolus Time/1 -> Subtract1/1
  Constant/1 -> Subtract1/2
  Subtract1/1 -> Overflow Counter/2(Upper Limit Of Counter), Relational Operator/2

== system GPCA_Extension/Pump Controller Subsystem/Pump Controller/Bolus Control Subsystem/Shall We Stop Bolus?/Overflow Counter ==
  Keep Running : Inport
  Upper Limit Of Counter : Inport  Port=2  OutDataType=sfix(16)  OutScaling=2^0
  Add : Sum  Orientation=left  OutDataType=sfix(16)  OutScaling=2^-10
  Constant : Constant  Value=0  OutDataType=sfix(16)  OutScaling=2^0
  Constant1 : Constant  Orientation=left  OutDataType=sfix(16)  OutScaling=2^0
  Counter : UnitDelay
  Logical Operator : Logic  AllPortsSameDT=off  OutDataTypeMode=boolean
  Update counter : Switch  Threshold=1  OutDataType=sfix(16)  OutScaling=2^0
  Value of Counter Less Than Threshold : RelationalOperator  Operator=<  LogicOutDataTypeMode=boolean
  Out1 : Outport
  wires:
  Add/1 -> Update counter/1
  Constant1/1 -> Add/1
  Counter/1 -> Add/2, Value of Counter Less Than Threshold/1
  Update counter/1 -> Counter/1, Out1/1
  Upper Limit Of Counter/1 -> Value of Counter Less Than Threshold/2
  Constant/1 -> Update counter/3
  Keep Running/1 -> Logical Operator/1
  Value of Counter Less Than Threshold/1 -> Logical Operator/2
  Logical Operator/1 -> Update counter/2
